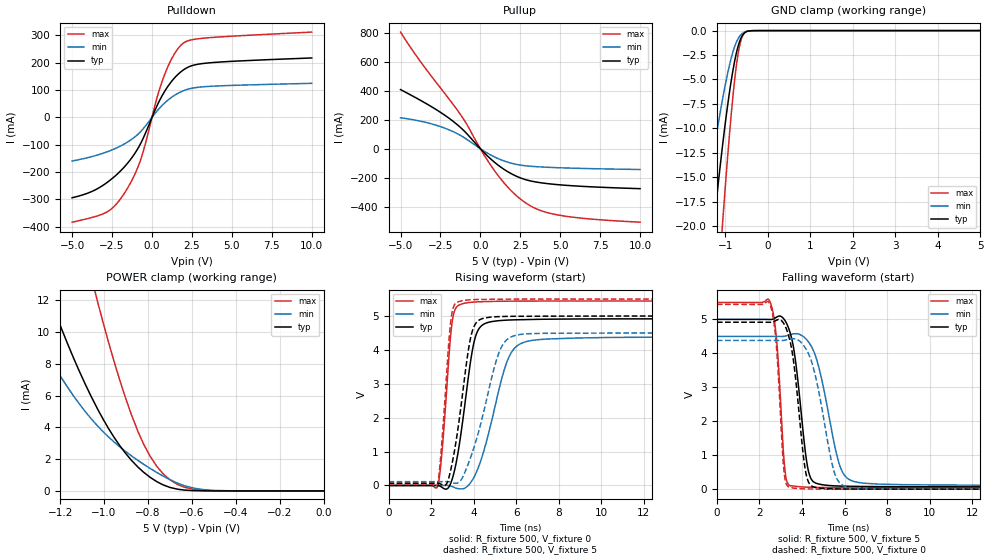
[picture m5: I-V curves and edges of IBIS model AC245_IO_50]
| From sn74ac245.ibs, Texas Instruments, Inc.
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[Model]   AC245_IO_50
Model_type  I/O
Vinl=1.35
Vinh=3.85
Enable   Active-Low
Vref =   0
Rref =   500
Cref =   50p
Vmeas =   2.5
| variable   typ   min   max
C_comp   6.92pF   6.31pF   8.03pF
| C_pullup   12.50pF   7.20pF   18.22pF
| C_pulldown   8.73pF   7.25pF   10.90pF
| C_tri-state   6.92pF   6.31pF   8.03pF
[Temperature Range]   40   100   -40
| Ambient temperature   25   85   -40
[Voltage range]   5   4.5   5.5
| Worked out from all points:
|   slope of the pulldown table from 0 to 0.75 V, typ, clamps not added: 8.23 ohm
|   slope of the pullup table from 0 to 0.75 V, typ, clamps not added: 9.31 ohm
|   GND clamp passes 1 mA (typ) near -0.66 V on its own axis
|   POWER clamp passes 1 mA (typ) near -0.80 V on its own axis
|   rising waveform, R_fixture 500, V_fixture 0: 20-80 % time 656ps typ, 1.08ns min, 382ps max; typ from 0 V to 4.92 V
|   falling waveform, R_fixture 500, V_fixture 5: 20-80 % time 524ps typ, 865ps min, 316ps max; typ from 5 V to 0.068 V
|   rising waveform, R_fixture 500, V_fixture 5: 20-80 % time 650ps typ, 1.09ns min, 368ps max; typ from 0.068 V to 5 V
|   falling waveform, R_fixture 500, V_fixture 0: 20-80 % time 499ps typ, 802ps min, 309ps max; typ from 4.92 V to 0 V
[GND Clamp]
| AC245_IO_50
|   Voltage   I(typ)   I(min)   I(max)
-5V       -257.6mA   -168.5mA   -326.6mA
-1.555V   -33mA      -20.85mA   -52.14mA
-1.505V   -30.55mA   -19.27mA   -48.61mA
-1.3V     -21.11mA   -13.12mA   -34.54mA
-1.25V    -18.97mA   -11.72mA   -31.23mA
-1.075V   -12.02mA   -7.192mA   -20.19mA
-1.055V   -11.29mA   -6.717mA   -18.99mA
-895mV    -6.015mA   -3.35mA    -10.12mA
-765mV    -2.74mA    -1.424mA   -4.358mA
-665mV    -1.098mA   -573.1uA   -1.518mA
-545mV    -209.6uA   -135.1uA   -215.6uA
5V        95.62nA    30.48uA    872nA
[POWER Clamp]
| AC245_IO_50
|   Voltage   I(typ)   I(min)   I(max)
-5V       307.3mA    212.4mA    474.5mA
-1.41V    18.74mA    12.56mA    36.85mA
-1.38V    17.45mA    11.72mA    34.58mA
-1.26V    12.61mA    8.625mA    25.99mA
-1.06V    5.976mA    4.561mA    13.55mA
-1.03V    5.163mA    4.094mA    11.92mA
-930mV    2.876mA    2.792mA    7.033mA
-845mV    1.49mA     1.91mA     3.717mA
-790mV    853uA      1.412mA    2.173mA
-700mV    219.2uA    708.8uA    695.5uA
-550mV    5.632uA    85.11uA    35.96uA
-84.45fV  95.62nA    5.578nA    1.326uA
[Pulldown]
| AC245_IO_50
|   Voltage   I(typ)   I(min)   I(max)
-5V       -293.7mA   -159.3mA   -383mA
-3.775V   -271mA     -143.3mA   -366mA
-2.79V    -236.8mA   -125.3mA   -344.4mA
-2.24V    -210.6mA   -112.1mA   -317.2mA
-1.62V    -173.6mA   -93.21mA   -267.2mA
-700mV    -94.19mA   -51.12mA   -153mA
310mV     42.12mA    23.14mA    71.14mA
790mV     94.99mA    52.74mA    156.8mA
1.355V    140.8mA    78.81mA    227.4mA
1.915V    171.6mA    96.32mA    269.6mA
3.475V    199.1mA    113.2mA    291.2mA
10V       217.6mA    124.7mA    312.1mA
[Pullup]
| AC245_IO_50
|   Voltage   I(typ)   I(min)   I(max)
-5V       407.1mA    213.1mA    803.2mA
-3.73V    331.9mA    189mA      596.8mA
-1.745V   191.9mA    119.5mA    311mA
-935mV    113.5mA    70.59mA    183.3mA
120mV     -14.11mA   -8.809mA   -22.35mA
885mV     -93.23mA   -56.6mA    -151.2mA
1.7V      -157.3mA   -92.23mA   -262.6mA
2.515V    -201.2mA   -113mA     -347.1mA
3.52V     -229.9mA   -123.7mA   -414.7mA
4.755V    -246.6mA   -130.4mA   -454.1mA
6.77V     -261.5mA   -136.8mA   -482.8mA
10V       -275.1mA   -143.1mA   -506mA
[Ramp]
| AC245_IO_50
| variable   typ   min   max
dV/dt_r   3.01/6.75E-10   2.69/1.11E-09   3.31/3.90E-10
dV/dt_f   3.02/5.44E-10   2.68/8.85E-10   3.33/3.31E-10
R_load = 500
[Rising Waveform]
| AC245_IO_50
R_fixture =   500
C_fixture =   0
L_fixture =   0
V_fixture =   0
V_fixture_min = 0
V_fixture_max = 0
|   Time   V(typ)   V(min)   V(max)
0s        32.92nV    7.046nV    244.4nV
2.31ns    1.387mV    -106.5uV   -23.14mV
2.51ns    -52.49mV   205uV      967.2mV
3.005ns   215.4mV    -33.08mV   4.881V
3.65ns    2.695V     -53.84mV   5.386V
3.99ns    4.144V     212.6mV    5.41V
4.31ns    4.675V     683.1mV    5.421V
5.63ns    4.881V     3.745V     5.438V
6.755ns   4.898V     4.281V     5.441V
50ns      4.917V     4.381V     5.442V
[Falling Waveform]
| AC245_IO_50
R_fixture =   500
C_fixture =   0
L_fixture =   0
V_fixture =   5
V_fixture_min = 4.5
V_fixture_max = 5.5
|   Time   V(typ)   V(min)   V(max)
0s        5V         4.5V       5.5V
2.51ns    4.998V     4.5V       5.499V
2.815ns   5.07V      4.499V     4.337V
3.2ns     4.966V     4.508V     553.5mV
3.475ns   4.533V     4.557V     98.61mV
4.285ns   581.7mV    4.353V     58.15mV
4.985ns   127.9mV    3.066V     50.26mV
5.84ns    90.48mV    588.1mV    46.66mV
6.9ns     79.32mV    176.1mV    44.96mV
50ns      68.27mV    112.4mV    43.77mV
[Rising Waveform]
| AC245_IO_50
R_fixture =   500
C_fixture =   0
L_fixture =   0
V_fixture =   5
V_fixture_min = 4.5
V_fixture_max = 5.5
|   Time   V(typ)   V(min)   V(max)
0s        68.27mV    112.4mV    43.77mV
2.29ns    69.96mV    112.3mV    28.55mV
2.465ns   39.99mV    112.5mV    953mV
2.945ns   520.2mV    96.03mV    4.939V
3.495ns   2.775V     255mV      5.454V
3.835ns   4.286V     786.9mV    5.478V
4.11ns    4.791V     1.311V     5.486V
5.225ns   4.983V     3.968V     5.496V
6.17ns    4.992V     4.454V     5.499V
50ns      5V         4.5V       5.5V
[Falling Waveform]
| AC245_IO_50
R_fixture =   500
C_fixture =   0
L_fixture =   0
V_fixture =   0
V_fixture_min = 0
V_fixture_max = 0
|   Time   V(typ)   V(min)   V(max)
0s        4.917V     4.381V     5.442V
2.49ns    4.915V     4.381V     5.445V
2.785ns   4.972V     4.38V      4.293V
3.17ns    4.849V     4.385V     437.4mV
3.51ns    4.139V     4.429V     40.45mV
4.075ns   920.6mV    4.236V     10.62mV
4.3ns     215.6mV    3.992V     6.788mV
5.52ns    8.519mV    496.4mV    1.404mV
6.29ns    3.076mV    43.72mV    674.8uV
50ns      42.51nV    292.8nV    344.2nV
